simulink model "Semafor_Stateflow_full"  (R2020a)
settings: Solver=VariableStepAuto  StartTime=0.0  StopTime=inf  RelTol=1e-3

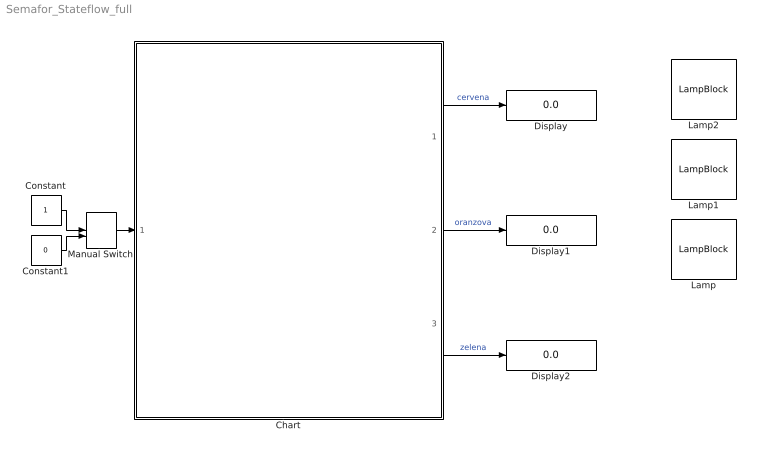
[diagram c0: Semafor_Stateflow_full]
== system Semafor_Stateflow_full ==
  Chart : Stateflow chart  TreatAsAtomicUnit=on
  Constant : Constant
  Constant1 : Constant  Value=0
  Display : Display
  Display1 : Display
  Display2 : Display
  Lamp : LampBlock  LabelPosition=Hide
  Lamp1 : LampBlock  LabelPosition=Hide
  Lamp2 : LampBlock  LabelPosition=Hide
  Manual Switch : ManualSwitch  CurrentSetting=0
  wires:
  Chart/1(cervena) -> Display/1  "cervena"
  Chart/2(oranzova) -> Display1/1  "oranzova"
  Chart/3(zelena) -> Display2/1  "zelena"
  Manual Switch/1 -> Chart/1(ZAP)
  Constant/1 -> Manual Switch/1
  Constant1/1 -> Manual Switch/2

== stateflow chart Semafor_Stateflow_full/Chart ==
  state Zapnuto
    state Volno
      entry:
      oranzova = 0;
      cervena = 0;
      zelena = 1;
    state Pripravse
      entry:
      oranzova = 1;
    state Pozor
      entry:
      zelena = 0;
      oranzova = 1;
    state Stuj
      entry:
      oranzova = 0;
      cervena = 1;
    Pripravse -> Volno : after(2,sec)
    Volno -> Pozor : after(5,sec)
    Stuj -> Pripravse : after(5,sec)
    (default) -> Pozor
    Pozor -> Stuj : after(2,sec)
  state Vypnuto
    state Svit
      entry:
      oranzova = 1;
    state Zhasni
      entry:
      oranzova = 0;
    (default) -> Svit : {cervena = 0; zelena = 0;}
    Zhasni -> Svit : after(1,sec)
    Svit -> Zhasni : after(1,sec)
  Zapnuto -> Vypnuto : [ZAP == 0]
  Vypnuto -> Zapnuto : [ZAP == 1]
  (default) -> Vypnuto
  data: cervena output =0; oranzova output =0; zelena output =0; ZAP input
